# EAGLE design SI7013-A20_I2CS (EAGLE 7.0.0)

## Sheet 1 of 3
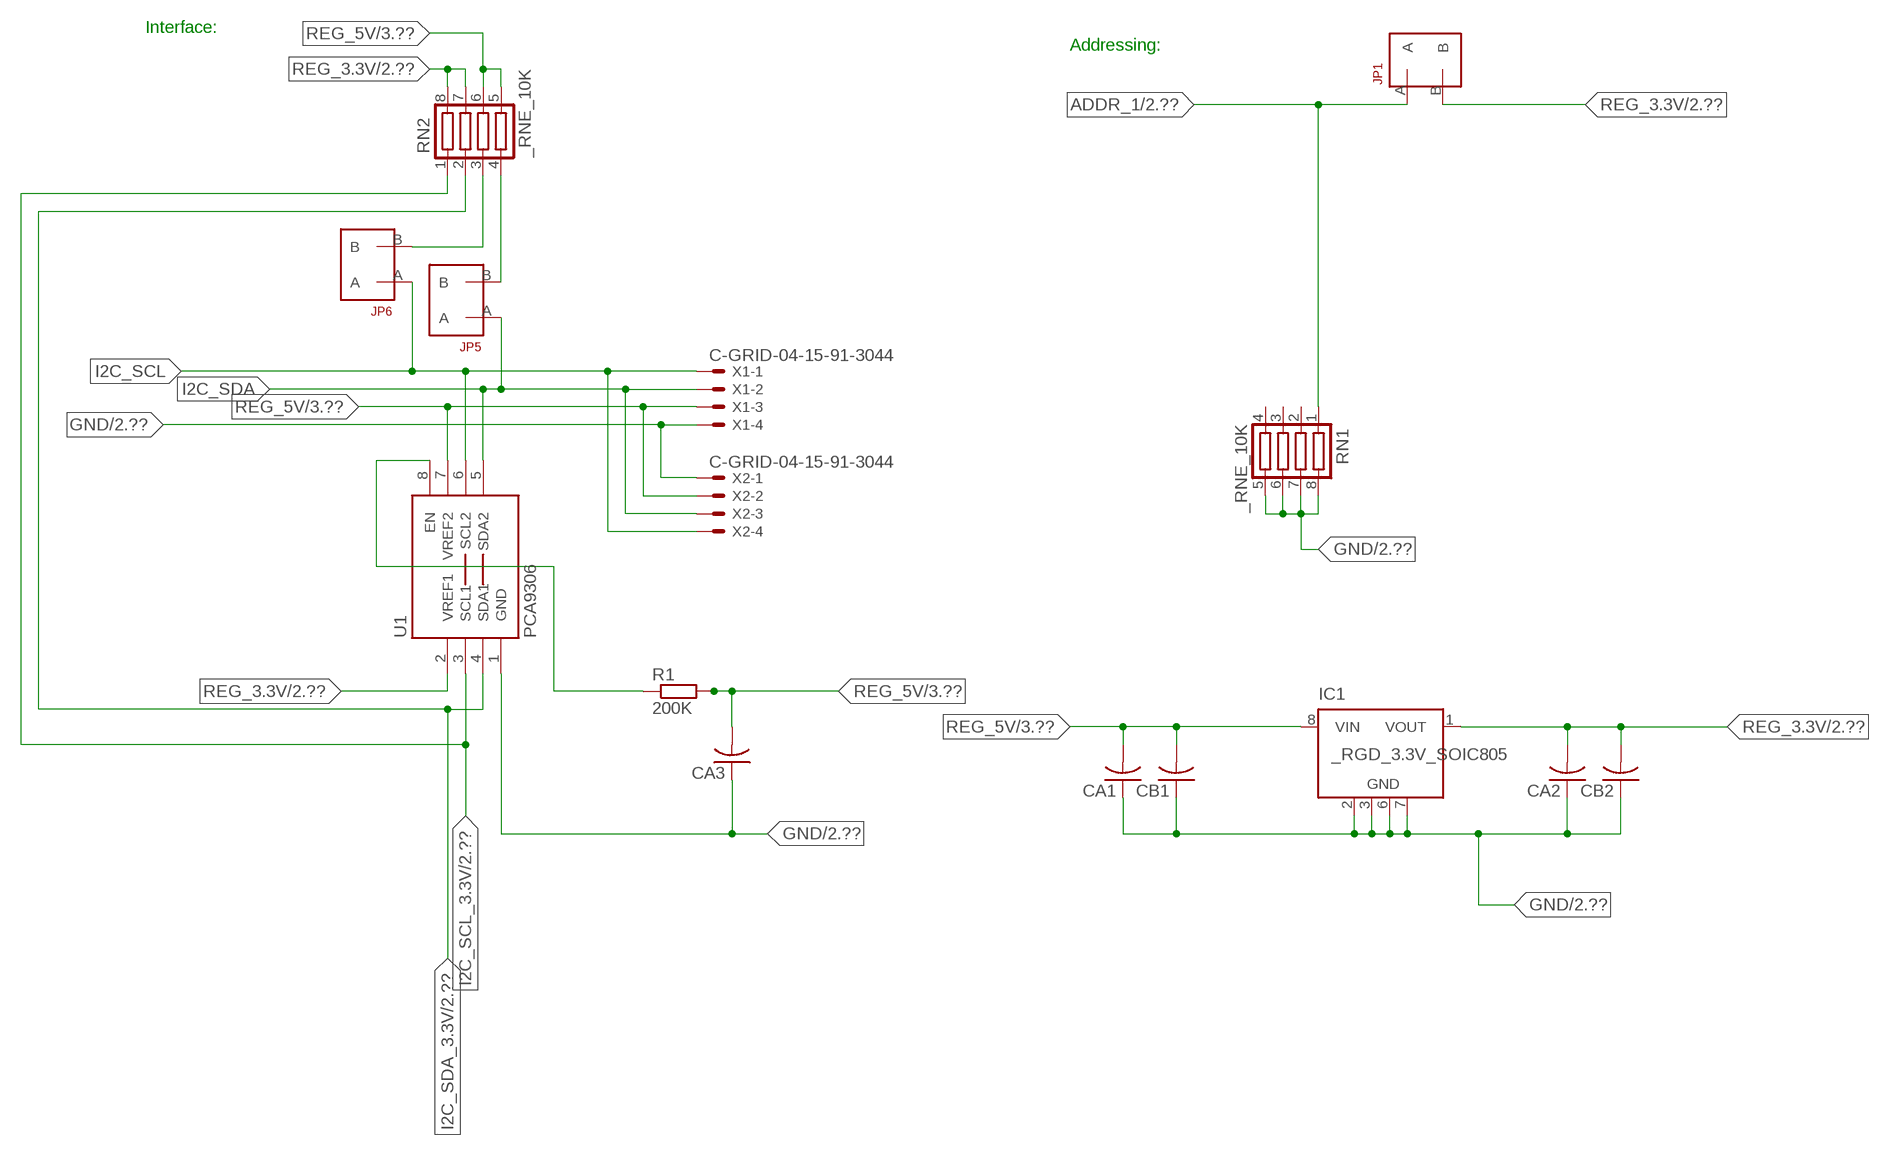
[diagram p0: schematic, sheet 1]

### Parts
CA1  CC1206KRX7R9BB104  [.1UF]
CA2  CC1206KRX7R9BB104  [.1UF]
CA3  CC1206KRX7R9BB104  [.1UF]
CB1  TMK316F106ZL-TC1206K  [TMK316F106ZL-T]
CB2  TMK316F106ZL-TC1206K  [TMK316F106ZL-T]
IC1  _RGD_3.3V_SOIC805  [_RGC_3.3V_SOIC8]
JP1  JUMPER_1X2_2MM  [JUMPER_1X2_2MM]
JP5  JUMPER_1X2_2MM  [JUMPER_1X2_2MM]
JP6  JUMPER_1X2_2MM  [JUMPER_1X2_2MM]
R1  200K  RESISTOR_SMT-0603  [R603]
RN1  _RNE_10K  [RNE]
RN2  _RNE_10K  [RNE]
U1  PCA9306  PCA9306_NCD  [PSOP-8]
X1  C-GRID-04-15-91-3044  [15-91-04]
X2  C-GRID-04-15-91-3044  [15-91-04]

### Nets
ADDR_1: JP1.A RN1.1 ; also sheet 2
GND: CA1.1 CA2.1 CA3.1 CB1.1 CB2.1 IC1.2(GND) IC1.3(GND) IC1.6(GND) IC1.7(GND) RN1.5 RN1.6 RN1.7 RN1.8 U1.1(GND) X1.4 X2.1 ; also sheet 2,3
I2C_SCL: JP6.A U1.6(SCL2) X1.1 X2.4
I2C_SCL_3.3V: RN2.1 U1.3(SCL1) ; also sheet 2
I2C_SDA: JP5.A U1.5(SDA2) X1.2 X2.3
I2C_SDA_3.3V: RN2.2 U1.4(SDA1) ; also sheet 2
N$1: JP6.B RN2.3
N$2: JP5.B RN2.4
N$27: R1.1 U1.8(EN)
REG_3.3V: CA2.2 CB2.2 IC1.1(VOUT) JP1.B RN2.7 RN2.8 U1.2(VREF1) ; also sheet 2
REG_5V: CA1.2 CA3.2 CB1.2 IC1.8(VIN) R1.2 RN2.5 RN2.6 U1.7(VREF2) X1.3 X2.2 ; also sheet 3
Unconnected: IC1.4(NC) IC1.5(NC) RN1.2 RN1.3 RN1.4

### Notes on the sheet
- Interface:
- Addressing:

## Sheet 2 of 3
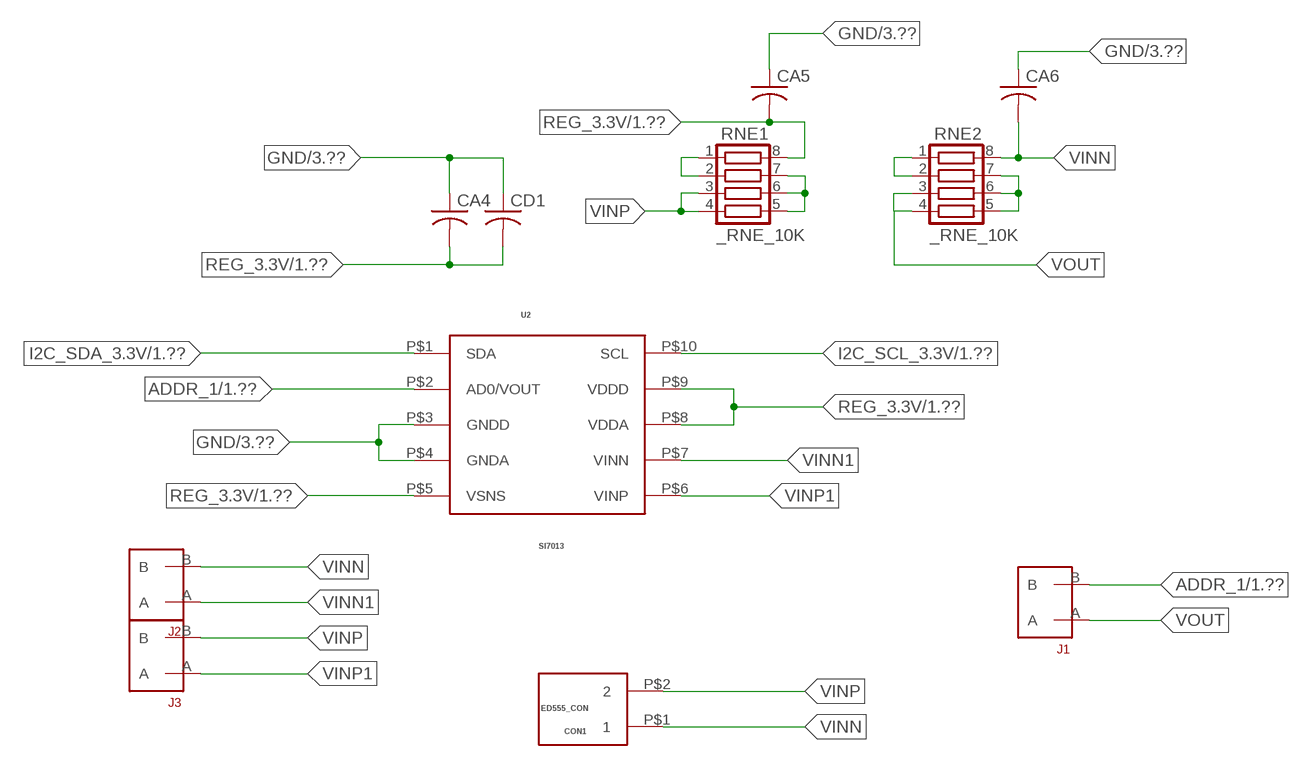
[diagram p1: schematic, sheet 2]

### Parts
CA4  _CA_.10UF_50VC1206K  [_CA_.1UF_50V]
CA5  _CA_.10UF_50VC1206K  [_CA_.1UF_50V]
CA6  _CA_.10UF_50VC1206K  [_CA_.1UF_50V]
CD1  _CD_10NF_50VC1206K  [_CD_10NF_50V]
CON1  ED555_CON  [ED555_CON]
J1  JUMPER_1X2_2MM  [JUMPER_1X2_2MM]
J2  JUMPER_1X2_2MM  [JUMPER_1X2_2MM]
J3  JUMPER_1X2_2MM  [JUMPER_1X2_2MM]
RNE1  _RNE_10K  [RNE]
RNE2  _RNE_10K  [RNE]
U2  SI7013  [SI7013]

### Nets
ADDR_1: J1.B U2.P$2(AD0/VOUT) ; also sheet 1
GND: CA4.1 CA5.1 CA6.1 CD1.1 U2.P$3(GNDD) U2.P$4(GNDA) ; also sheet 1,3
I2C_SCL_3.3V: U2.P$10(SCL) ; also sheet 1
I2C_SDA_3.3V: U2.P$1(SDA) ; also sheet 1
N$14: RNE1.1 RNE1.2
N$16: RNE1.5 RNE1.6 RNE1.7
N$18: RNE2.1 RNE2.2
N$19: RNE2.5 RNE2.6 RNE2.7
REG_3.3V: CA4.2 CA5.2 CD1.2 RNE1.8 U2.P$5(VSNS) U2.P$8(VDDA) U2.P$9(VDDD) ; also sheet 1
VINN: CA6.2 CON1.P$1 J2.B RNE2.8
VINN1: J2.A U2.P$7(VINN)
VINP: CON1.P$2 J3.B RNE1.3 RNE1.4
VINP1: J3.A U2.P$6(VINP)
VOUT: J1.A RNE2.3 RNE2.4

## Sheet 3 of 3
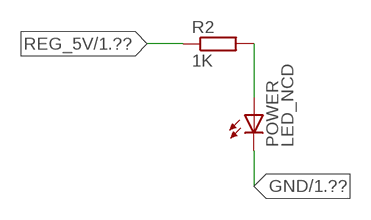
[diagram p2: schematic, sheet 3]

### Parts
POWER  LED_NCD  [CHIPLED_0603]
R2  1K  RESISTOR_SMT-0402  [R402]

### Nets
GND: POWER.C ; also sheet 1,2
N$4: POWER.A R2.2
REG_5V: R2.1 ; also sheet 1

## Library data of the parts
CA1-CA3 = NCD_ULTIMATE_LIBRARY:CC1206KRX7R9BB104: Capacitor CA .1uF 50V SMT C1206K CC1206KRX7R9BB104
CA4-CA6 = NCD_ULTIMATE_LIBRARY:_CA_.10UF_50V: Capacitor .1uF SMT
CB1 CB2 = NCD_ULTIMATE_LIBRARY:TMK316F106ZL-T: Capacitor CB 10uF SMT 1206 TMK316F106ZL-T
CD1 = NCD_ULTIMATE_LIBRARY:_CD_10NF_50V: Capacitor 10nF SMT
CON1 = NCD_ULTIMATE_bhaskar:ED555_CON: Digikey ED1514-ND/ ED555/2DS NCD CON
IC1 = NCD_ULTIMATE_LIBRARY:_RGD_3.3V_SOIC8: Regulator Linear 3.3V Chip Positive VOLTAGE REGULATOR Digikey 497-1199-2-ND/L78L33ACD13TR
J1-J3 JP1 JP5 JP6 = NCD_ULTIMATE_CONNECTORS:JUMPER_1X2_2MM
POWER = NCD_ULTIMATE_LIBRARY:LED_NCD: LED Digikey 754-1132-2-ND/APT2012SRCPRV
R1 R2 = NCD_ULTIMATE_LIBRARY:RESISTOR_SMT: NCD Resistor
RN1 RN2 RNE1 RNE2 = NCD_ULTIMATE_LIBRARY:_RNE_10K: Resistor Array RNE SMT 10K x 4 Single Resistor Source: http://www.ctscorp.com/components/Datasheets/CTSChipArrayDs.pdf Digikey 742C083103JPTR-ND/742C083103JP; OC_FARNELL: unknown; OC_NEWARK: unknown
U1 = NCD_ULTIMATE_LIBRARY:PCA9306_NCD: NCD Bidirectional I2C level shifter. NOT compatible with all available part number pinout schemes- DOUBLE CHECK!!!; PROD_ID: IC-10023
U2 = NCD_ULTIMATE_bhaskar:SI7013: http://www.silabs.com/products/sensors/humidity-sensors/Pages/si7013-20-21.aspx
X1 X2 = NCD_ULTIMATE_CONNECTORS:C-GRID-04: CONNECTOR 4-Pos I2C wire to board 2.54 mm (0.100") pitch header Digikey WM1342-ND/0015912045; OC_FARNELL: unknown; OC_NEWARK: unknown

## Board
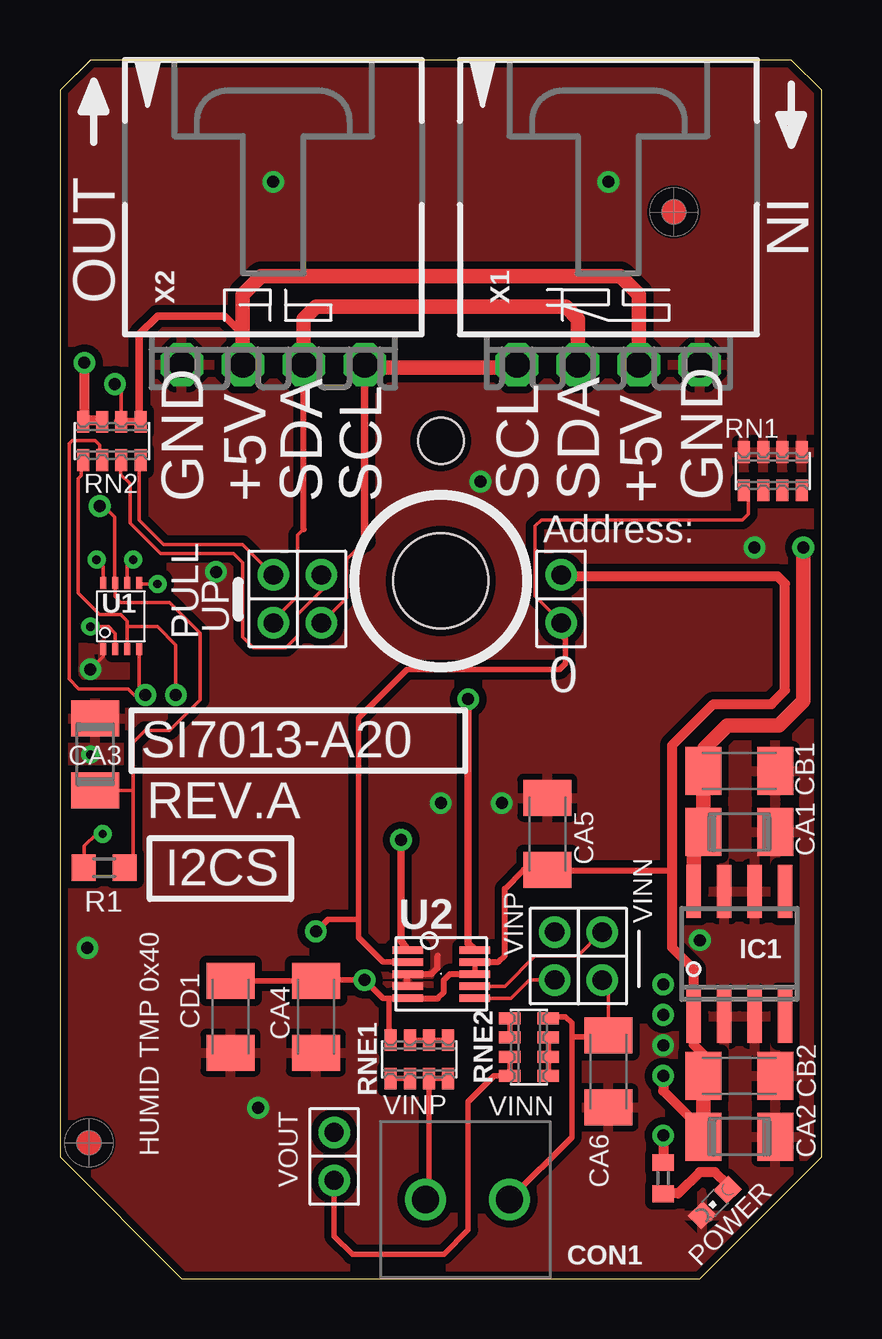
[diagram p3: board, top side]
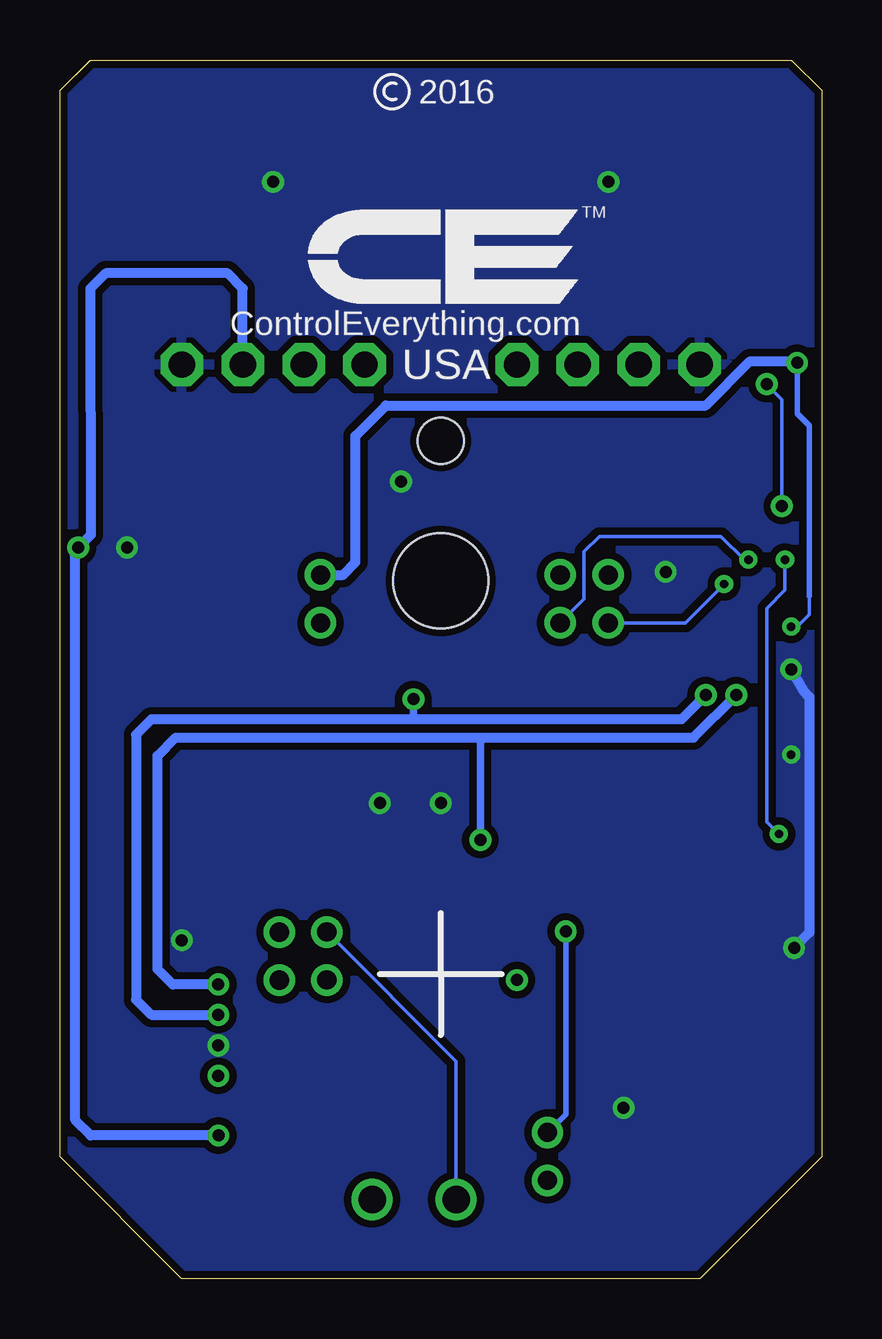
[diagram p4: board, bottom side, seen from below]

Size 31.75 x 50.8 mm. Coordinates in mm from the lower left corner, seen from the top.
Outline: 32 segments
Copper layers (1*16): Top 0.035mm / dielectric 1.5mm / Bottom 0.035mm
Design rules "default": minimum track width 5mil, minimum drill 24mil, track to track 5mil, track to pad 5mil, pad to pad 5mil, via to via 5mil, smd to smd 5mil, copper to edge 10mil, drill to drill 8mil, minimum pad ring 10mil, minimum via ring 8mil, stop-mask expansion 2mil, vias tented up to drill 0mil, thermal gap 10mil
Holes 3.96 mm at 15.88,29.08
Holes 1.91 mm at 15.88,34.93

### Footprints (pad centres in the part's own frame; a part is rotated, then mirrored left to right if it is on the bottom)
.1UF = smd 1.5 x 2: 1 -1.5,0; 2 1.5,0
_CA_.1UF_50V = smd 1.5 x 2: 1 -1.5,0; 2 1.5,0
TMK316F106ZL-T = smd 1.5 x 2: 1 -1.5,0; 2 1.5,0
_CD_10NF_50V = smd 1.5 x 2: 1 -1.5,0; 2 1.5,0
ED555_CON = drill 1.143: P$1 0,3.5; P$2 0,0
_RGC_3.3V_SOIC8 = smd 0.6 x 2.2: 1 -1.905,-2.6; 2 -0.635,-2.6; 3 0.635,-2.6; 4 1.905,-2.6; 5 1.905,2.6; 6 0.635,2.6; 7 -0.635,2.6; 8 -1.905,2.6
JUMPER_1X2_2MM = drill 0.8: A 0,2; B 0,0
CHIPLED_0603 = smd 0.8 x 0.876: A 0,-0.75; C 0,0.75
R603 = smd 1 x 1.1: 1 -0.85,0; 2 0.85,0
R402 = smd 0.7 x 0.9: 1 -0.65,0; 2 0.65,0
RNE = smd 0.5 x 0.9: 1 -1.2,-0.8; 2 -0.4,-0.8; 3 0.4,-0.8; 4 1.2,-0.8; 5 1.2,0.8; 6 0.4,0.8; 7 -0.4,0.8; 8 -1.2,0.8
PSOP-8 = smd 0.25 x 0.5: 1 -0.73,-1.37; 2 -0.23,-1.37; 3 0.27,-1.37; 4 0.77,-1.37; 5 0.77,1.38; 6 0.27,1.38; 7 -0.23,1.38; 8 -0.73,1.38
SI7013 = smd 1.27 x 0.3: P$1 -1,1; P$2 -1,0.5; P$3 -1,0; P$4 -1,-0.5; P$5 -1,-1; P$6 1.8,-1; P$7 1.8,-0.5; P$8 1.8,0; P$9 1.8,0.5; P$10 1.8,1
15-91-04 = drill 1.1 pad 1.778 octagon: 1 -3.81,-7.62; 2 -1.27,-7.62; 3 1.27,-7.62; 4 3.81,-7.62

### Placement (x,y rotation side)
CA1  28.32,18.62 180 top
CA2  28.32,5.92 180 top
CA3  1.46,21.86 270 top
CA4  10.67,10.92 90 top
CA5  20.32,18.54 270 top
CA6  22.86,8.64 90 top
CB1  28.32,21.16 180 top
CB2  28.32,8.46 180 top
CD1  7.11,10.92 90 top
CON1  15.24,3.3 270 top
IC1  28.32,13.54 0 top
J1  11.43,6.1 180 top
J2  22.61,12.45 0 top
J3  20.62,14.45 180 top
JP1  20.89,29.34 180 top
JP5  8.89,29.34 180 top
JP6  10.9,29.34 180 top
POWER  27.3,3.18 135 top
R1  1.84,17.13 0 top
R2  25.15,4.19 270 top
RN1  29.72,33.66 0 top
RN2  2.16,34.93 0 top
RNE1  14.99,9.14 0 top
RNE2  19.56,9.65 270 top
U1  2.54,27.61 0 top
U2  15.49,12.7 0 top
U$5  [VISION_REF10]  1.21,5.66 90 top
U$28  [VISION_REF10]  25.59,44.46 90 top
X1  22.86,45.72 0 top
X2  8.89,45.72 0 top

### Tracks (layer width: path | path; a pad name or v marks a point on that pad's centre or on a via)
ADDR_1  (via drill 0.5)
  Top 0.152: JP1.A 20.89,27.37 19.81,28.45 19.81,31.37 20.07,31.62 28.45,31.62 28.7,31.88 28.7,32.78 RN1.1
  Top 0.229: U2.P$2 13.46,13.21 12.45,14.22 12.45,14.99 | 12.45,14.99 12.45,23.37 14.48,25.4 20.83,25.4 21.08,25.65 21.08,26.67 20.89,26.86 JP1.A | v10.67,14.48 11.18,14.99 12.45,14.99
  Bottom 0.229: J1.B 10.67,6.86 v10.67,14.48
GND  (via drill 0.35, 0.5)
  Top 0.152: CA3.1 1.52,23.42 1.52,23.62 | v1.27,25.4 1.81,25.94 U1.1
  Top 0.254: U2.P$3 U2.P$4 14.48,12.22 14.48,12.7 15.49,12.7 15.75,12.95 15.75,13.46
  Bottom 0.406: v1.27,25.4 0.76,24.51 0.51,24.26 0.51,14.43 v1.15,13.79
  other vias: 8.89,45.72 22.86,45.72 25.15,9.73 17.53,33.22 26.67,14.11 6.5,29.46 28.96,30.48 15.88,19.82 18.42,19.82 8.26,7.12 1.27,21.84
  pour Bottom (isolate 0.305): -0.64,5.08 -0.64,49.53 1.27,51.44 30.48,51.44 32.38,49.53 32.38,5.08 26.67,-0.63 5.08,-0.63
  pour Top (isolate 0.305): 4.45,-1.27 -1.27,4.45 -1.27,50.17 0.64,52.07 31.11,52.07 33.02,50.17 33.02,4.45 27.3,-1.27
I2C_SCL  (via drill 0.35)
  Top 0.152: 12.7,30.73 11.94,29.97 11.94,28.38 JP6.A | v3.05,29.97 2.81,29.73 U1.6
  Top 0.305: 12.7,30.73 X2.4
  Top 0.406: X2.4 12.7,37.97 | 19.05,37.97 X1.1
  Top 0.61: 12.7,37.97 19.05,37.97
  Bottom 0.152: JP6.A 9.91,28.33 9.91,30.3 9.27,30.94 4.19,30.94 3.23,29.97 v3.05,29.97
I2C_SCL_3.3V  (via drill 0.5)
  Top 0.152: RN2.1 0.89,34.07 0.89,33.48 0.77,33.35 0.77,28.59 1.67,27.69 2.54,27.69 2.81,27.42 2.81,27.18 | 2.81,27.18 U1.3 | v4.83,24.33 v4.83,24.34 4.83,26.42 4.06,27.18 2.81,27.18
  Top 0.305: U2.P$10 17.02,13.98 v17.02,24.16
  Bottom 0.305: v17.02,24.16 17.02,23.32
  Bottom 0.406: v4.83,24.33 5.84,23.32 17.02,23.32 27.94,23.32 28.58,22.68 28.58,11.63 27.94,11 v25.15,11
I2C_SDA  (via drill 0.35)
  Top 0.152: JP5.A 8.89,27.44 9.91,28.45 9.91,30.99 10.16,31.24 | U1.5 3.34,28.96 v4.06,28.96
  Top 0.254: 10.16,31.24 10.16,31.25 X2.3
  Top 0.61: X2.3 10.16,40.01 10.67,40.51 21.09,40.51 21.59,40.01 X1.2
  Bottom 0.152: v4.06,28.96 5.68,27.34 JP5.A
I2C_SDA_3.3V  (via drill 0.5)
  Top 0.152: RN2.2 1.65,34.14 1.65,34.75 1.46,34.94 0.51,34.94 0.38,34.81 0.38,26.37 0.38,26.36 0.38,24.99 0.79,24.59 2.85,24.59 3.1,24.33 v3.56,24.33 3.31,24.58 U1.4
  Top 0.305: U2.P$1 14.22,14.08 v14.22,18.29
  Bottom 0.305: v14.22,18.29 14.22,22.56
  Bottom 0.406: v25.15,12.27 27.05,12.27 27.69,12.9 27.69,21.79 26.93,22.56 14.22,22.56 5.34,22.56 v3.56,24.33
N$1
  Top 0.152: JP6.B 10.92,29.31 10.92,28.7 9.91,27.69 9.91,26.8 9.42,26.31 8.06,26.31 7.62,26.75 7.62,29.84 7.24,30.23 4.19,30.23 2.92,31.5 2.92,33.15 2.54,33.53 2.54,34.1 RN2.3
  Top 0.305: 2.54,34.02 RN2.3
N$2
  Top 0.152: JP5.B 7.62,30.61 4.32,30.61 3.3,31.62 3.3,34.07 RN2.4
  Top 0.305: 3.37,33.88 RN2.4
N$4
  Top 0.406: POWER.A 27.84,3.92 27.3,4.45 26.67,4.45 25.78,3.56 25.16,3.56 R2.2
N$14
  Top 0.229: RNE1.2 RNE1.1
N$16
  Top 0.229: RNE1.5 RNE1.6 RNE1.7
N$18
  Top 0.229: RNE2.1 18.8,10.81 18.8,10.67 18.76,10.63 RNE2.2
N$19
  Top 0.229: RNE2.5 RNE2.6 RNE2.7
N$27  (via drill 0.35)
  Top 0.152: R1.1 1.02,17.16 1.02,18.03 1.52,18.54 v1.78,18.54 | v1.52,29.97 1.81,29.69 U1.8
  Bottom 0.152: v1.78,18.54 2.29,19.05 2.29,27.94 1.52,28.7 v1.52,29.97
REG_3.3V  (via drill 0.35, 0.5)
  Top 0.152: v1.27,27.18 2.03,27.18 2.31,26.9 U1.2
  Top 0.229: U2.P$9 U2.P$8 | U2.P$5 13.72,11.68 | CD1.2 CA4.2 10.69,12.45 v12.7,12.45 13.46,11.68 13.72,11.68 | RNE1.8 13.72,10.52 13.72,11.68
  Top 0.254: U2.P$5 14.51,11.68 15.75,11.68 16,11.94 16,12.45 16.26,12.7 U2.P$8 | U2.P$9 17.3,13.21 18.29,13.21 18.54,13.46 18.54,16.26 19.33,17.04 CA5.2 20.34,17.02 25.53,17.02
  Top 0.406: CB2.2 26.82,9.35 26.42,9.75 26.42,10.36 | v25.15,8.46 25.15,7.82 26.42,6.55 26.82,6.55 | IC1.1 26.42,12.9 25.53,13.79 25.53,17.02 25.53,22.24 27.24,23.95 29.66,23.95 30.23,24.52 30.23,28.97 29.91,29.29 20.95,29.29 JP1.B | 26.52,5.62 CA2.2 | v1.02,38.18 1.02,35.78 | 1.02,35.78 RN2.8 | 1.02,35.78 1.71,35.78 RN2.7
  Top 0.61: CB2.2 26.82,6.55 CA2.2 | 26.42,10.36 IC1.1
  Bottom 0.152: 0.51,28.45 0.51,27.69 1.02,27.18 v1.27,27.18
  Bottom 0.229: 0.51,28.45 0.51,35.56 1.02,36.07 v1.02,38.18 | v12.7,12.45 12.95,12.7 | 24.82,8.46 v25.15,8.46
  Bottom 0.406: v1.02,38.18 1.08,38.24 2.99,38.24 4.83,36.4 18.16,36.4 19.43,35.13 19.43,29.87 19.94,29.34 JP1.B
REG_5V  (via drill 0.5)
  Top 0.152: RN2.6 2.56,37.01 v2.29,37.29 | R1.2 3.05,17.49 3.05,20.36 | 3.05,20.36 3.05,22.35 3.56,22.86 4.57,22.86 5.84,24.13 5.84,26.92 4.57,28.19 2.54,28.19 2.31,28.43 U1.7 2.29,29.01 2.29,31.75 1.83,32.21 v1.65,32.21 | CA3.2 3.05,20.36
  Top 0.305: 7.62,39.37 7.5,39.37 | 2.42,35.74 RN2.6 RN2.5 3.31,35.8 3.31,39.37 4.07,40.13 6.86,40.13 7.62,39.37 | X2.2 7.62,39.37
  Top 0.406: v25.15,5.97 R2.1
  Top 0.61: X2.2 7.62,41.02 8.38,41.78 23.37,41.78 24.13,41.02 X1.3 | IC1.8 26.42,18.21 CA1.2 CB1.2 26.86,21.2 26.86,22.11 27.82,23.06 29.98,23.06 30.99,24.08 v30.99,30.48
  Bottom 0.152: v1.65,32.21 1.65,36.65 v2.29,37.29
  Bottom 0.406: X1.3 24.13,41.28 24.77,41.91 29.84,41.91 30.48,41.27 30.47,31 v30.99,30.48 31.11,30.36 31.11,6.6 30.48,5.97 v25.15,5.97
VINN
  Top 0.152: J2.B 22.86,12.19 CA6.2
  Top 0.229: 20.32,10.89 RNE2.8 20.43,10.92 21.08,10.92 21.34,10.67 21.34,10.09 | CA6.2 22.81,10.09 21.34,10.09 | CON1.P$1 21.34,5.9 21.34,10.09
VINN1
  Top 0.152: U2.P$7 17.3,12.19 18.54,12.19 19.81,13.46 21.59,13.46 22.57,14.45 J2.A
VINP
  Top 0.229: RNE1.4 RNE1.3 15.39,3.45 CON1.P$2
  Bottom 0.152: J3.B 15.24,9.07 CON1.P$2
VINP1
  Top 0.152: U2.P$6 17.31,11.68 18.8,11.68 19.57,12.45 J3.A
VOUT
  Top 0.229: RNE2.3 RNE2.4 18.1,8.45 17.02,7.37 17.02,2.03 16,1.02 12.19,1.02 11.43,1.78 J1.A

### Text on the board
tNames: IN | OUT | GND | +5V | SDA | SCL | SCL | SDA | +5V | GND | Address: | PULL | UP | 0 | SI7013-A20 | REV.A | VINN | I2CS | HUMID TMP 0x40 | VINP | VINN | VINP | VOUT
bNames: 2016 | TM | ControlEverything.com | USA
